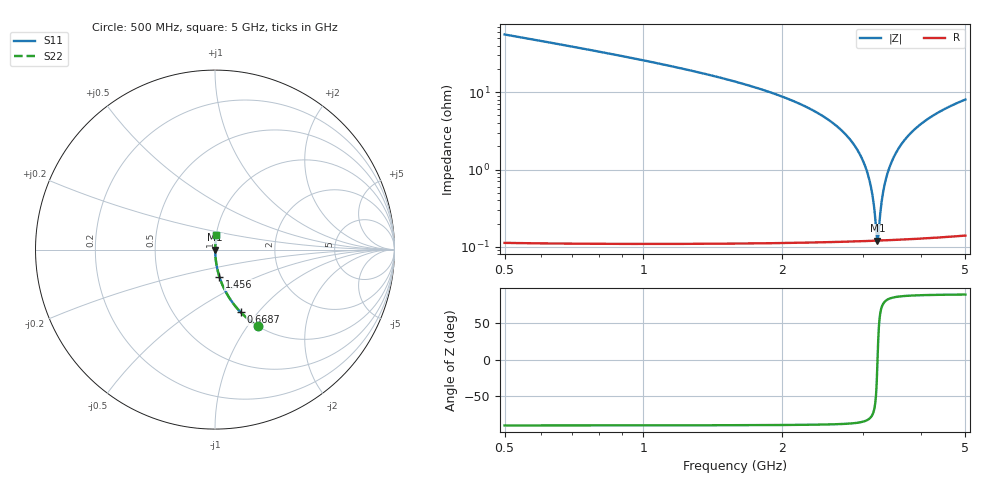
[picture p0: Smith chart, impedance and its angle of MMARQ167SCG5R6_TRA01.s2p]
! MMARQ167SCG5R6_TRA01  S-PARAMETER MODEL  ( General Type )
! Model Generated by TAIYO YUDEN Corporation (http://www.ty-top.com)
! Version 1.0
! TAIYO YUDEN Control No. 150305
! Copyright(c) 2015 TAIYO YUDEN CO.,LTD. All Rights Reserved.
! Product Description (link to TY-COMPAS)
! https://ds.yuden.co.jp/TYCOMPAS/or/detail?pn=MMARQ167SCG5R6CTRA01&u=M
! Products Name : Multilayer Ceramic Capacitors
! Characteristics :
!  Capacitance : 5.6 pF , Rated Voltage : 250V , TCC : CG / C0G
!  Case Size : 1.6 x 0.8 / 0.063 x 0.031 [mm/inch] , Thickness : 0.7 / 0.028 [mm/inch]
!  (Conditions: Temperature = 25 degC , DC Bias Current/Voltage = 0A / 0V)
! External Node Assignments :
!  1  o---| |---o  2
! GND o---------o GND
! Frequency Range : 500MHz  -  5GHz  [ 401 STEP ]
# MHz S RI R 50
! Freq[MHz].  S11 Real  S11 Imag  S21 Real  S21 Imag  S12 Real  S12 Imag  S22 Real  S22 Imag
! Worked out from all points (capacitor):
!   401 points, 500 MHz to 5 GHz, reference 50 ohm
!   read as one part in series: C = 5.57 pF near 522.5 MHz
!   lowest |Z| = 120 mohm at 3.223 GHz (marker M1)
!   series resonance near 3.223 GHz, so ESL is about 440 pH
!   S11 on the Smith chart (normalised r, x): 500 MHz: 1.00, -1.12; 668.8 MHz: 1.00, -0.82; 1.456 GHz: 1.00, -0.31; 5 GHz: 1.00, +0.16
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500  0.2379 -0.4248  0.7621 0.4248  0.7621 0.4248  0.2379 -0.4248
668.75  0.144 -0.3498  0.856 0.3498  0.856 0.3498  0.144 -0.3498
1253.75  0.0371 -0.1861  0.9629 0.1861  0.9629 0.1861  0.0371 -0.1861
1456.25  0.0248 -0.1522  0.9752 0.1522  0.9752 0.1522  0.0248 -0.1522
2007.5  0.00863 -0.0863  0.9914 0.0863  0.9914 0.0863  0.00863 -0.0863
2446.25  0.00358 -0.0493  0.9964 0.0493  0.9964 0.0493  0.00358 -0.0493
2750  0.00196 -0.0282  0.998 0.0282  0.998 0.0282  0.00196 -0.0282
2930  0.00146 -0.0169  0.9985 0.0169  0.9985 0.0169  0.00146 -0.0169
3065  0.00127 -0.00891  0.9987 0.00891  0.9987 0.00891  0.00127 -0.00891
3143.75  0.00121 -0.00442  0.9988 0.00442  0.9988 0.00442  0.00121 -0.00442
3166.25  0.00121 -0.00316  0.9988 0.00316  0.9988 0.00316  0.00121 -0.00316
3200  0.0012 -0.00128  0.9988 0.00128  0.9988 0.00128  0.0012 -0.00128
3222.5  0.0012 -4.28e-05  0.9988 4.28e-05  0.9988 4.28e-05  0.0012 -4.28e-05
3245  0.0012 0.00119  0.9988 -0.00119  0.9988 -0.00119  0.0012 0.00119
3290  0.00122 0.00363  0.9988 -0.00363  0.9988 -0.00363  0.00122 0.00363
3335  0.00125 0.00603  0.9988 -0.00603  0.9988 -0.00603  0.00125 0.00603
3402.5  0.00131 0.00958  0.9987 -0.00958  0.9987 -0.00958  0.00131 0.00958
3503.75  0.00145 0.0148  0.9986 -0.0148  0.9986 -0.0148  0.00145 0.0148
3627.5  0.00168 0.0209  0.9983 -0.0209  0.9983 -0.0209  0.00168 0.0209
3796.25  0.0021 0.0291  0.9979 -0.0291  0.9979 -0.0291  0.0021 0.0291
4257.5  0.00379 0.0497  0.9962 -0.0497  0.9962 -0.0497  0.00379 0.0497
5000  0.00779 0.0797  0.9922 -0.0797  0.9922 -0.0797  0.00779 0.0797
